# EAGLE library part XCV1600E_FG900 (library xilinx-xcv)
xcv1600e_fg900 edit this description Auto generated by make-symbol-device-package-bsdl.ulp Rev. 26 Source: xcv1600e_fg900.bsd
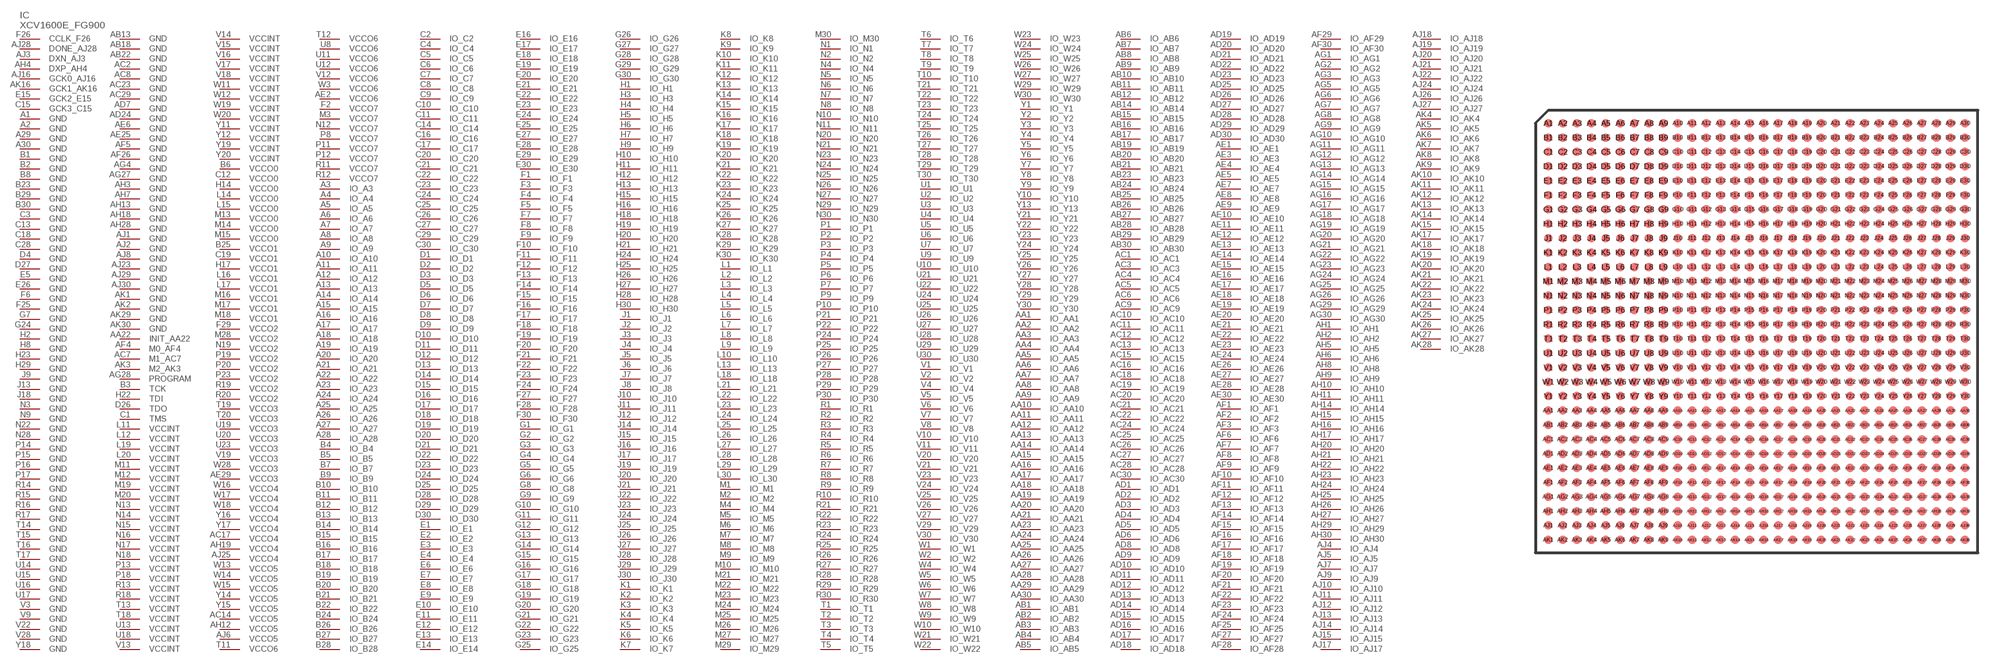
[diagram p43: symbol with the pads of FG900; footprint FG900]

Designator prefix IC

## XCV1600E_FG900 (OC_FARNELL: unknown; OC_NEWARK: unknown)  [FG900]
A1  GND  pwr
A2  GND  pwr
A3  IO_A3
A4  IO_A4
A5  IO_A5
A6  IO_A6
A7  IO_A7
A8  IO_A8
A9  IO_A9
A10  IO_A10
A11  IO_A11
A12  IO_A12
A13  IO_A13
A14  IO_A14
A15  IO_A15
A16  IO_A16
A17  IO_A17
A18  IO_A18
A19  IO_A19
A20  IO_A20
A21  IO_A21
A22  IO_A22
A23  IO_A23
A24  IO_A24
A25  IO_A25
A26  IO_A26
A27  IO_A27
A28  IO_A28
A29  GND  pwr
A30  GND  pwr
AA1  IO_AA1
AA2  IO_AA2
AA3  IO_AA3
AA4  IO_AA4
AA5  IO_AA5
AA6  IO_AA6
AA7  IO_AA7
AA8  IO_AA8
AA9  IO_AA9
AA10  IO_AA10
AA11  IO_AA11
AA12  IO_AA12
AA13  IO_AA13
AA14  IO_AA14
AA15  IO_AA15
AA16  IO_AA16
AA17  IO_AA17
AA18  IO_AA18
AA19  IO_AA19
AA20  IO_AA20
AA21  IO_AA21
AA22  INIT_AA22
AA23  IO_AA23
AA24  IO_AA24
AA25  IO_AA25
AA26  IO_AA26
AA27  IO_AA27
AA28  IO_AA28
AA29  IO_AA29
AA30  IO_AA30
AB1  IO_AB1
AB2  IO_AB2
AB3  IO_AB3
AB4  IO_AB4
AB5  IO_AB5
AB6  IO_AB6
AB7  IO_AB7
AB8  IO_AB8
AB9  IO_AB9
AB10  IO_AB10
AB11  IO_AB11
AB12  IO_AB12
AB13  GND  pwr
AB14  IO_AB14
AB15  IO_AB15
AB16  IO_AB16
AB17  IO_AB17
AB18  GND  pwr
AB19  IO_AB19
AB20  IO_AB20
AB21  IO_AB21
AB22  GND  pwr
AB23  IO_AB23
AB24  IO_AB24
AB25  IO_AB25
AB26  IO_AB26
AB27  IO_AB27
AB28  IO_AB28
AB29  IO_AB29
AB30  IO_AB30
AC1  IO_AC1
AC2  GND  pwr
AC3  IO_AC3
AC4  IO_AC4
AC5  IO_AC5
AC6  IO_AC6
AC7  M1_AC7  in
AC8  GND  pwr
AC9  IO_AC9
AC10  IO_AC10
AC11  IO_AC11
AC12  IO_AC12
AC13  IO_AC13
AC14  VCCO5  pwr
AC15  IO_AC15
AC16  IO_AC16
AC17  VCCO4  pwr
AC18  IO_AC18
AC19  IO_AC19
AC20  IO_AC20
AC21  IO_AC21
AC22  IO_AC22
AC23  GND  pwr
AC24  IO_AC24
AC25  IO_AC25
AC26  IO_AC26
AC27  IO_AC27
AC28  IO_AC28
AC29  GND  pwr
AC30  IO_AC30
AD1  IO_AD1
AD2  IO_AD2
AD3  IO_AD3
AD4  IO_AD4
AD5  IO_AD5
AD6  IO_AD6
AD7  GND  pwr
AD8  IO_AD8
AD9  IO_AD9
AD10  IO_AD10
AD11  IO_AD11
AD12  IO_AD12
AD13  IO_AD13
AD14  IO_AD14
AD15  IO_AD15
AD16  IO_AD16
AD17  IO_AD17
AD18  IO_AD18
AD19  IO_AD19
AD20  IO_AD20
AD21  IO_AD21
AD22  IO_AD22
AD23  IO_AD23
AD24  GND  pwr
AD25  IO_AD25
AD26  IO_AD26
AD27  IO_AD27
AD28  IO_AD28
AD29  IO_AD29
AD30  IO_AD30
AE1  IO_AE1
AE2  VCCO6  pwr
AE3  IO_AE3
AE4  IO_AE4
AE5  IO_AE5
AE6  GND  pwr
AE7  IO_AE7
AE8  IO_AE8
AE9  IO_AE9
AE10  IO_AE10
AE11  IO_AE11
AE12  IO_AE12
AE13  IO_AE13
AE14  IO_AE14
AE15  IO_AE15
AE16  IO_AE16
AE17  IO_AE17
AE18  IO_AE18
AE19  IO_AE19
AE20  IO_AE20
AE21  IO_AE21
AE22  IO_AE22
AE23  IO_AE23
AE24  IO_AE24
AE25  GND  pwr
AE26  IO_AE26
AE27  IO_AE27
AE28  IO_AE28
AE29  VCCO3  pwr
AE30  IO_AE30
AF1  IO_AF1
AF2  IO_AF2
AF3  IO_AF3
AF4  M0_AF4  in
AF5  GND  pwr
AF6  IO_AF6
AF7  IO_AF7
AF8  IO_AF8
AF9  IO_AF9
AF10  IO_AF10
AF11  IO_AF11
AF12  IO_AF12
AF13  IO_AF13
AF14  IO_AF14
AF15  IO_AF15
AF16  IO_AF16
AF17  IO_AF17
AF18  IO_AF18
AF19  IO_AF19
AF20  IO_AF20
AF21  IO_AF21
AF22  IO_AF22
AF23  IO_AF23
AF24  IO_AF24
AF25  IO_AF25
AF26  GND  pwr
AF27  IO_AF27
AF28  IO_AF28
AF29  IO_AF29
AF30  IO_AF30
AG1  IO_AG1
AG2  IO_AG2
AG3  IO_AG3
AG4  GND  pwr
AG5  IO_AG5
AG6  IO_AG6
AG7  IO_AG7
AG8  IO_AG8
AG9  IO_AG9
AG10  IO_AG10
AG11  IO_AG11
AG12  IO_AG12
AG13  IO_AG13
AG14  IO_AG14
AG15  IO_AG15
AG16  IO_AG16
AG17  IO_AG17
AG18  IO_AG18
AG19  IO_AG19
AG20  IO_AG20
AG21  IO_AG21
AG22  IO_AG22
AG23  IO_AG23
AG24  IO_AG24
AG25  IO_AG25
AG26  IO_AG26
AG27  GND  pwr
AG28  PROGRAM  in
AG29  IO_AG29
AG30  IO_AG30
AH1  IO_AH1
AH2  IO_AH2
AH3  GND  pwr
AH4  DXP_AH4  pas
AH5  IO_AH5
AH6  IO_AH6
AH7  GND  pwr
AH8  IO_AH8
AH9  IO_AH9
AH10  IO_AH10
AH11  IO_AH11
AH12  VCCO5  pwr
AH13  GND  pwr
AH14  IO_AH14
AH15  IO_AH15
AH16  IO_AH16
AH17  IO_AH17
AH18  GND  pwr
AH19  VCCO4  pwr
AH20  IO_AH20
AH21  IO_AH21
AH22  IO_AH22
AH23  IO_AH23
AH24  IO_AH24
AH25  IO_AH25
AH26  IO_AH26
AH27  IO_AH27
AH28  GND  pwr
AH29  IO_AH29
AH30  IO_AH30
AJ1  GND  pwr
AJ2  GND  pwr
AJ3  DXN_AJ3  pas
AJ4  IO_AJ4
AJ5  IO_AJ5
AJ6  VCCO5  pwr
AJ7  IO_AJ7
AJ8  GND  pwr
AJ9  IO_AJ9
AJ10  IO_AJ10
AJ11  IO_AJ11
AJ12  IO_AJ12
AJ13  IO_AJ13
AJ14  IO_AJ14
AJ15  IO_AJ15
AJ16  GCK0_AJ16  in
AJ17  IO_AJ17
AJ18  IO_AJ18
AJ19  IO_AJ19
AJ20  IO_AJ20
AJ21  IO_AJ21
AJ22  IO_AJ22
AJ23  GND  pwr
AJ24  IO_AJ24
AJ25  VCCO4  pwr
AJ26  IO_AJ26
AJ27  IO_AJ27
AJ28  DONE_AJ28
AJ29  GND  pwr
AJ30  GND  pwr
AK1  GND  pwr
AK2  GND  pwr
AK3  M2_AK3  in
AK4  IO_AK4
AK5  IO_AK5
AK6  IO_AK6
AK7  IO_AK7
AK8  IO_AK8
AK9  IO_AK9
AK10  IO_AK10
AK11  IO_AK11
AK12  IO_AK12
AK13  IO_AK13
AK14  IO_AK14
AK15  IO_AK15
AK16  GCK1_AK16  in
AK17  IO_AK17
AK18  IO_AK18
AK19  IO_AK19
AK20  IO_AK20
AK21  IO_AK21
AK22  IO_AK22
AK23  IO_AK23
AK24  IO_AK24
AK25  IO_AK25
AK26  IO_AK26
AK27  IO_AK27
AK28  IO_AK28
AK29  GND  pwr
AK30  GND  pwr
B1  GND  pwr
B2  GND  pwr
B3  TCK  in
B4  IO_B4
B5  IO_B5
B6  VCCO0  pwr
B7  IO_B7
B8  GND  pwr
B9  IO_B9
B10  IO_B10
B11  IO_B11
B12  IO_B12
B13  IO_B13
B14  IO_B14
B15  IO_B15
B16  IO_B16
B17  IO_B17
B18  IO_B18
B19  IO_B19
B20  IO_B20
B21  IO_B21
B22  IO_B22
B23  GND  pwr
B24  IO_B24
B25  VCCO1  pwr
B26  IO_B26
B27  IO_B27
B28  IO_B28
B29  GND  pwr
B30  GND  pwr
C1  TMS  in
C2  IO_C2
C3  GND  pwr
C4  IO_C4
C5  IO_C5
C6  IO_C6
C7  IO_C7
C8  IO_C8
C9  IO_C9
C10  IO_C10
C11  IO_C11
C12  VCCO0  pwr
C13  GND  pwr
C14  IO_C14
C15  GCK3_C15  in
C16  IO_C16
C17  IO_C17
C18  GND  pwr
C19  VCCO1  pwr
C20  IO_C20
C21  IO_C21
C22  IO_C22
C23  IO_C23
C24  IO_C24
C25  IO_C25
C26  IO_C26
C27  IO_C27
C28  GND  pwr
C29  IO_C29
C30  IO_C30
D1  IO_D1
D2  IO_D2
D3  IO_D3
D4  GND  pwr
D5  IO_D5
D6  IO_D6
D7  IO_D7
D8  IO_D8
D9  IO_D9
D10  IO_D10
D11  IO_D11
D12  IO_D12
D13  IO_D13
D14  IO_D14
D15  IO_D15
D16  IO_D16
D17  IO_D17
D18  IO_D18
D19  IO_D19
D20  IO_D20
D21  IO_D21
D22  IO_D22
D23  IO_D23
D24  IO_D24
D25  IO_D25
D26  TDO  out
D27  GND  pwr
D28  IO_D28
D29  IO_D29
D30  IO_D30
E1  IO_E1
E2  IO_E2
E3  IO_E3
E4  IO_E4
E5  GND  pwr
E6  IO_E6
E7  IO_E7
E8  IO_E8
E9  IO_E9
E10  IO_E10
E11  IO_E11
E12  IO_E12
E13  IO_E13
E14  IO_E14
E15  GCK2_E15  in
E16  IO_E16
E17  IO_E17
E18  IO_E18
E19  IO_E19
E20  IO_E20
E21  IO_E21
E22  IO_E22
E23  IO_E23
E24  IO_E24
E25  IO_E25
E26  GND  pwr
E27  IO_E27
E28  IO_E28
E29  IO_E29
E30  IO_E30
F1  IO_F1
F2  VCCO7  pwr
F3  IO_F3
F4  IO_F4
F5  IO_F5
F6  GND  pwr
F7  IO_F7
F8  IO_F8
F9  IO_F9
F10  IO_F10
F11  IO_F11
F12  IO_F12
F13  IO_F13
F14  IO_F14
F15  IO_F15
F16  IO_F16
F17  IO_F17
F18  IO_F18
F19  IO_F19
F20  IO_F20
F21  IO_F21
F22  IO_F22
F23  IO_F23
F24  IO_F24
F25  GND  pwr
F26  CCLK_F26
F27  IO_F27
F28  IO_F28
F29  VCCO2  pwr
F30  IO_F30
G1  IO_G1
G2  IO_G2
G3  IO_G3
G4  IO_G4
G5  IO_G5
G6  IO_G6
G7  GND  pwr
G8  IO_G8
G9  IO_G9
G10  IO_G10
G11  IO_G11
G12  IO_G12
G13  IO_G13
G14  IO_G14
G15  IO_G15
G16  IO_G16
G17  IO_G17
G18  IO_G18
G19  IO_G19
G20  IO_G20
G21  IO_G21
G22  IO_G22
G23  IO_G23
G24  GND  pwr
G25  IO_G25
G26  IO_G26
G27  IO_G27
G28  IO_G28
G29  IO_G29
G30  IO_G30
H1  IO_H1
H2  GND  pwr
H3  IO_H3
H4  IO_H4
H5  IO_H5
H6  IO_H6
H7  IO_H7
H8  GND  pwr
H9  IO_H9
H10  IO_H10
H11  IO_H11
H12  IO_H12
H13  IO_H13
H14  VCCO0  pwr
H15  IO_H15
H16  IO_H16
H17  VCCO1  pwr
H18  IO_H18
H19  IO_H19
H20  IO_H20
H21  IO_H21
H22  TDI  in
H23  GND  pwr
H24  IO_H24
H25  IO_H25
H26  IO_H26
H27  IO_H27
H28  IO_H28
H29  GND  pwr
H30  IO_H30
J1  IO_J1
J2  IO_J2
J3  IO_J3
J4  IO_J4
J5  IO_J5
J6  IO_J6
J7  IO_J7
J8  IO_J8
J9  GND  pwr
J10  IO_J10
J11  IO_J11
J12  IO_J12
J13  GND  pwr
J14  IO_J14
J15  IO_J15
J16  IO_J16
J17  IO_J17
J18  GND  pwr
J19  IO_J19
J20  IO_J20
J21  IO_J21
J22  IO_J22
J23  IO_J23
J24  IO_J24
J25  IO_J25
J26  IO_J26
J27  IO_J27
J28  IO_J28
J29  IO_J29
J30  IO_J30
K1  IO_K1
K2  IO_K2
K3  IO_K3
K4  IO_K4
K5  IO_K5
K6  IO_K6
K7  IO_K7
K8  IO_K8
K9  IO_K9
K10  IO_K10
K11  IO_K11
K12  IO_K12
K13  IO_K13
K14  IO_K14
K15  IO_K15
K16  IO_K16
K17  IO_K17
K18  IO_K18
K19  IO_K19
K20  IO_K20
K21  IO_K21
K22  IO_K22
K23  IO_K23
K24  IO_K24
K25  IO_K25
K26  IO_K26
K27  IO_K27
K28  IO_K28
K29  IO_K29
K30  IO_K30
L1  IO_L1
L2  IO_L2
L3  IO_L3
L4  IO_L4
L5  IO_L5
L6  IO_L6
L7  IO_L7
L8  IO_L8
L9  IO_L9
L10  IO_L10
L11  VCCINT  pwr
L12  VCCINT  pwr
L13  IO_L13
L14  VCCO0  pwr
L15  VCCO0  pwr
L16  VCCO1  pwr
L17  VCCO1  pwr
L18  IO_L18
L19  VCCINT  pwr
L20  VCCINT  pwr
L21  IO_L21
L22  IO_L22
L23  IO_L23
L24  IO_L24
L25  IO_L25
L26  IO_L26
L27  IO_L27
L28  IO_L28
L29  IO_L29
L30  IO_L30
M1  IO_M1
M2  IO_M2
M3  VCCO7  pwr
M4  IO_M4
M5  IO_M5
M6  IO_M6
M7  IO_M7
M8  IO_M8
M9  IO_M9
M10  IO_M10
M11  VCCINT  pwr
M12  VCCINT  pwr
M13  VCCO0  pwr
M14  VCCO0  pwr
M15  VCCO0  pwr
M16  VCCO1  pwr
M17  VCCO1  pwr
M18  VCCO1  pwr
M19  VCCINT  pwr
M20  VCCINT  pwr
M21  IO_M21
M22  IO_M22
M23  IO_M23
M24  IO_M24
M25  IO_M25
M26  IO_M26
M27  IO_M27
M28  VCCO2  pwr
M29  IO_M29
M30  IO_M30
N1  IO_N1
N2  IO_N2
N3  GND  pwr
N4  IO_N4
N5  IO_N5
N6  IO_N6
N7  IO_N7
N8  IO_N8
N9  GND  pwr
N10  IO_N10
N11  IO_N11
N12  VCCO7  pwr
N13  VCCINT  pwr
N14  VCCINT  pwr
N15  VCCINT  pwr
N16  VCCINT  pwr
N17  VCCINT  pwr
N18  VCCINT  pwr
N19  VCCO2  pwr
N20  IO_N20
N21  IO_N21
N22  GND  pwr
N23  IO_N23
N24  IO_N24
N25  IO_N25
N26  IO_N26
N27  IO_N27
N28  GND  pwr
N29  IO_N29
N30  IO_N30
P1  IO_P1
P2  IO_P2
P3  IO_P3
P4  IO_P4
P5  IO_P5
P6  IO_P6
P7  IO_P7
P8  VCCO7  pwr
P9  IO_P9
P10  IO_P10
P11  VCCO7  pwr
P12  VCCO7  pwr
P13  VCCINT  pwr
P14  GND  pwr
P15  GND  pwr
P16  GND  pwr
P17  GND  pwr
P18  VCCINT  pwr
P19  VCCO2  pwr
P20  VCCO2  pwr
P21  IO_P21
P22  IO_P22
P23  VCCO2  pwr
P24  IO_P24
P25  IO_P25
P26  IO_P26
P27  IO_P27
P28  IO_P28
P29  IO_P29
P30  IO_P30
R1  IO_R1
R2  IO_R2
R3  IO_R3
R4  IO_R4
R5  IO_R5
R6  IO_R6
R7  IO_R7
R8  IO_R8
R9  IO_R9
R10  IO_R10
R11  VCCO7  pwr
R12  VCCO7  pwr
R13  VCCINT  pwr
R14  GND  pwr
R15  GND  pwr
R16  GND  pwr
R17  GND  pwr
R18  VCCINT  pwr
R19  VCCO2  pwr
R20  VCCO2  pwr
R21  IO_R21
R22  IO_R22
R23  IO_R23
R24  IO_R24
R25  IO_R25
R26  IO_R26
R27  IO_R27
R28  IO_R28
R29  IO_R29
R30  IO_R30
T1  IO_T1
T2  IO_T2
T3  IO_T3
T4  IO_T4
T5  IO_T5
T6  IO_T6
T7  IO_T7
T8  IO_T8
T9  IO_T9
T10  IO_T10
T11  VCCO6  pwr
T12  VCCO6  pwr
T13  VCCINT  pwr
T14  GND  pwr
T15  GND  pwr
T16  GND  pwr
T17  GND  pwr
T18  VCCINT  pwr
T19  VCCO3  pwr
T20  VCCO3  pwr
T21  IO_T21
T22  IO_T22
T23  IO_T23
T24  IO_T24
T25  IO_T25
T26  IO_T26
T27  IO_T27
T28  IO_T28
T29  IO_T29
T30  IO_T30
U1  IO_U1
U2  IO_U2
U3  IO_U3
U4  IO_U4
U5  IO_U5
U6  IO_U6
U7  IO_U7
U8  VCCO6  pwr
U9  IO_U9
U10  IO_U10
U11  VCCO6  pwr
U12  VCCO6  pwr
U13  VCCINT  pwr
U14  GND  pwr
U15  GND  pwr
U16  GND  pwr
U17  GND  pwr
U18  VCCINT  pwr
U19  VCCO3  pwr
U20  VCCO3  pwr
U21  IO_U21
U22  IO_U22
U23  VCCO3  pwr
U24  IO_U24
U25  IO_U25
U26  IO_U26
U27  IO_U27
U28  IO_U28
U29  IO_U29
U30  IO_U30
V1  IO_V1
V2  IO_V2
V3  GND  pwr
V4  IO_V4
V5  IO_V5
V6  IO_V6
V7  IO_V7
V8  IO_V8
V9  GND  pwr
V10  IO_V10
V11  IO_V11
V12  VCCO6  pwr
V13  VCCINT  pwr
V14  VCCINT  pwr
V15  VCCINT  pwr
V16  VCCINT  pwr
V17  VCCINT  pwr
V18  VCCINT  pwr
V19  VCCO3  pwr
V20  IO_V20
V21  IO_V21
V22  GND  pwr
V23  IO_V23
V24  IO_V24
V25  IO_V25
V26  IO_V26
V27  IO_V27
V28  GND  pwr
V29  IO_V29
V30  IO_V30
W1  IO_W1
W2  IO_W2
W3  VCCO6  pwr
W4  IO_W4
W5  IO_W5
W6  IO_W6
W7  IO_W7
W8  IO_W8
W9  IO_W9
W10  IO_W10
W11  VCCINT  pwr
W12  VCCINT  pwr
W13  VCCO5  pwr
W14  VCCO5  pwr
W15  VCCO5  pwr
W16  VCCO4  pwr
W17  VCCO4  pwr
W18  VCCO4  pwr
W19  VCCINT  pwr
W20  VCCINT  pwr
W21  IO_W21
W22  IO_W22
W23  IO_W23
W24  IO_W24
W25  IO_W25
W26  IO_W26
W27  IO_W27
W28  VCCO3  pwr
W29  IO_W29
W30  IO_W30
Y1  IO_Y1
Y2  IO_Y2
Y3  IO_Y3
Y4  IO_Y4
Y5  IO_Y5
Y6  IO_Y6
Y7  IO_Y7
Y8  IO_Y8
Y9  IO_Y9
Y10  IO_Y10
Y11  VCCINT  pwr
Y12  VCCINT  pwr
Y13  IO_Y13
Y14  VCCO5  pwr
Y15  VCCO5  pwr
Y16  VCCO4  pwr
Y17  VCCO4  pwr
Y18  GND  pwr
Y19  VCCINT  pwr
Y20  VCCINT  pwr
Y21  IO_Y21
Y22  IO_Y22
Y23  IO_Y23
Y24  IO_Y24
Y25  IO_Y25
Y26  IO_Y26
Y27  IO_Y27
Y28  IO_Y28
Y29  IO_Y29
Y30  IO_Y30

## Footprint FG900 (pad centres in mm)
xcv1000e_fg900_1532 edit this description Auto generated by make-symbol-device-package-bsdl.ulp Rev. 26 Source: xcv1000e_fg900_1532.bsd
smd 0.6 x 0.6: A1 -14.5,14.5; A2 -13.5,14.5; A3 -12.5,14.5; A4 -11.5,14.5; A5 -10.5,14.5; A6 -9.5,14.5; A7 -8.5,14.5; A8 -7.5,14.5; A9 -6.5,14.5; A10 -5.5,14.5; A11 -4.5,14.5; A12 -3.5,14.5; A13 -2.5,14.5; A14 -1.5,14.5; A15 -0.5,14.5; A16 0.5,14.5; A17 1.5,14.5; A18 2.5,14.5; A19 3.5,14.5; A20 4.5,14.5; A21 5.5,14.5; A22 6.5,14.5; A23 7.5,14.5; A24 8.5,14.5; A25 9.5,14.5; A26 10.5,14.5; A27 11.5,14.5; A28 12.5,14.5; A29 13.5,14.5; A30 14.5,14.5; AA1 -14.5,-5.5; AA2 -13.5,-5.5; AA3 -12.5,-5.5; AA4 -11.5,-5.5; AA5 -10.5,-5.5; AA6 -9.5,-5.5; AA7 -8.5,-5.5; AA8 -7.5,-5.5; AA9 -6.5,-5.5; AA10 -5.5,-5.5; AA11 -4.5,-5.5; AA12 -3.5,-5.5; AA13 -2.5,-5.5; AA14 -1.5,-5.5; AA15 -0.5,-5.5; AA16 0.5,-5.5; AA17 1.5,-5.5; AA18 2.5,-5.5; AA19 3.5,-5.5; AA20 4.5,-5.5; AA21 5.5,-5.5; AA22 6.5,-5.5; AA23 7.5,-5.5; AA24 8.5,-5.5; AA25 9.5,-5.5; AA26 10.5,-5.5; AA27 11.5,-5.5; AA28 12.5,-5.5; AA29 13.5,-5.5; AA30 14.5,-5.5; AB1 -14.5,-6.5; AB2 -13.5,-6.5; AB3 -12.5,-6.5; AB4 -11.5,-6.5; AB5 -10.5,-6.5; AB6 -9.5,-6.5; AB7 -8.5,-6.5; AB8 -7.5,-6.5; AB9 -6.5,-6.5; AB10 -5.5,-6.5; AB11 -4.5,-6.5; AB12 -3.5,-6.5; AB13 -2.5,-6.5; AB14 -1.5,-6.5; AB15 -0.5,-6.5; AB16 0.5,-6.5; AB17 1.5,-6.5; AB18 2.5,-6.5; AB19 3.5,-6.5; AB20 4.5,-6.5; AB21 5.5,-6.5; AB22 6.5,-6.5; AB23 7.5,-6.5; AB24 8.5,-6.5; AB25 9.5,-6.5; AB26 10.5,-6.5; AB27 11.5,-6.5; AB28 12.5,-6.5; AB29 13.5,-6.5; AB30 14.5,-6.5; AC1 -14.5,-7.5; AC2 -13.5,-7.5; AC3 -12.5,-7.5; AC4 -11.5,-7.5; AC5 -10.5,-7.5; AC6 -9.5,-7.5; AC7 -8.5,-7.5; AC8 -7.5,-7.5; AC9 -6.5,-7.5; AC10 -5.5,-7.5; AC11 -4.5,-7.5; AC12 -3.5,-7.5; AC13 -2.5,-7.5; AC14 -1.5,-7.5; AC15 -0.5,-7.5; AC16 0.5,-7.5; AC17 1.5,-7.5; AC18 2.5,-7.5; AC19 3.5,-7.5; AC20 4.5,-7.5; AC21 5.5,-7.5; AC22 6.5,-7.5; AC23 7.5,-7.5; AC24 8.5,-7.5; AC25 9.5,-7.5; AC26 10.5,-7.5; AC27 11.5,-7.5; AC28 12.5,-7.5; AC29 13.5,-7.5; AC30 14.5,-7.5; AD1 -14.5,-8.5; AD2 -13.5,-8.5; AD3 -12.5,-8.5; AD4 -11.5,-8.5; AD5 -10.5,-8.5; AD6 -9.5,-8.5; AD7 -8.5,-8.5; AD8 -7.5,-8.5; AD9 -6.5,-8.5; AD10 -5.5,-8.5; AD11 -4.5,-8.5; AD12 -3.5,-8.5; AD13 -2.5,-8.5; AD14 -1.5,-8.5; AD15 -0.5,-8.5; AD16 0.5,-8.5; AD17 1.5,-8.5; AD18 2.5,-8.5; AD19 3.5,-8.5; AD20 4.5,-8.5; AD21 5.5,-8.5; AD22 6.5,-8.5; AD23 7.5,-8.5; AD24 8.5,-8.5; AD25 9.5,-8.5; AD26 10.5,-8.5; AD27 11.5,-8.5; AD28 12.5,-8.5; AD29 13.5,-8.5; AD30 14.5,-8.5; AE1 -14.5,-9.5; AE2 -13.5,-9.5; AE3 -12.5,-9.5; AE4 -11.5,-9.5; AE5 -10.5,-9.5; AE6 -9.5,-9.5; AE7 -8.5,-9.5; AE8 -7.5,-9.5; AE9 -6.5,-9.5; AE10 -5.5,-9.5; AE11 -4.5,-9.5; AE12 -3.5,-9.5; AE13 -2.5,-9.5; AE14 -1.5,-9.5; AE15 -0.5,-9.5; AE16 0.5,-9.5; AE17 1.5,-9.5; AE18 2.5,-9.5; AE19 3.5,-9.5; AE20 4.5,-9.5; AE21 5.5,-9.5; AE22 6.5,-9.5; AE23 7.5,-9.5; AE24 8.5,-9.5; AE25 9.5,-9.5; AE26 10.5,-9.5; AE27 11.5,-9.5; AE28 12.5,-9.5; AE29 13.5,-9.5; AE30 14.5,-9.5; AF1 -14.5,-10.5; AF2 -13.5,-10.5; AF3 -12.5,-10.5; AF4 -11.5,-10.5; AF5 -10.5,-10.5; AF6 -9.5,-10.5; AF7 -8.5,-10.5; AF8 -7.5,-10.5; AF9 -6.5,-10.5; AF10 -5.5,-10.5; AF11 -4.5,-10.5; AF12 -3.5,-10.5; AF13 -2.5,-10.5; AF14 -1.5,-10.5; AF15 -0.5,-10.5; AF16 0.5,-10.5; AF17 1.5,-10.5; AF18 2.5,-10.5; AF19 3.5,-10.5; AF20 4.5,-10.5; AF21 5.5,-10.5; AF22 6.5,-10.5; AF23 7.5,-10.5; AF24 8.5,-10.5; AF25 9.5,-10.5; AF26 10.5,-10.5; AF27 11.5,-10.5; AF28 12.5,-10.5; AF29 13.5,-10.5; AF30 14.5,-10.5; AG1 -14.5,-11.5; AG2 -13.5,-11.5; AG3 -12.5,-11.5; AG4 -11.5,-11.5; AG5 -10.5,-11.5; AG6 -9.5,-11.5; AG7 -8.5,-11.5; AG8 -7.5,-11.5; AG9 -6.5,-11.5; AG10 -5.5,-11.5; AG11 -4.5,-11.5; AG12 -3.5,-11.5; AG13 -2.5,-11.5; AG14 -1.5,-11.5; AG15 -0.5,-11.5; AG16 0.5,-11.5; AG17 1.5,-11.5; AG18 2.5,-11.5; AG19 3.5,-11.5; AG20 4.5,-11.5; AG21 5.5,-11.5; AG22 6.5,-11.5; AG23 7.5,-11.5; AG24 8.5,-11.5; AG25 9.5,-11.5; AG26 10.5,-11.5; AG27 11.5,-11.5; AG28 12.5,-11.5; AG29 13.5,-11.5; AG30 14.5,-11.5; AH1 -14.5,-12.5; AH2 -13.5,-12.5; AH3 -12.5,-12.5; AH4 -11.5,-12.5; AH5 -10.5,-12.5; AH6 -9.5,-12.5; AH7 -8.5,-12.5; AH8 -7.5,-12.5; AH9 -6.5,-12.5; AH10 -5.5,-12.5; AH11 -4.5,-12.5; AH12 -3.5,-12.5; AH13 -2.5,-12.5; AH14 -1.5,-12.5; AH15 -0.5,-12.5; AH16 0.5,-12.5; AH17 1.5,-12.5; AH18 2.5,-12.5; AH19 3.5,-12.5; AH20 4.5,-12.5; AH21 5.5,-12.5; AH22 6.5,-12.5; AH23 7.5,-12.5; AH24 8.5,-12.5; AH25 9.5,-12.5; AH26 10.5,-12.5; AH27 11.5,-12.5; AH28 12.5,-12.5; AH29 13.5,-12.5; AH30 14.5,-12.5; AJ1 -14.5,-13.5; AJ2 -13.5,-13.5; AJ3 -12.5,-13.5; AJ4 -11.5,-13.5; AJ5 -10.5,-13.5; AJ6 -9.5,-13.5; AJ7 -8.5,-13.5; AJ8 -7.5,-13.5; AJ9 -6.5,-13.5; AJ10 -5.5,-13.5; AJ11 -4.5,-13.5; AJ12 -3.5,-13.5; AJ13 -2.5,-13.5; AJ14 -1.5,-13.5; AJ15 -0.5,-13.5; AJ16 0.5,-13.5; AJ17 1.5,-13.5; AJ18 2.5,-13.5; AJ19 3.5,-13.5; AJ20 4.5,-13.5; AJ21 5.5,-13.5; AJ22 6.5,-13.5; AJ23 7.5,-13.5; AJ24 8.5,-13.5; AJ25 9.5,-13.5; AJ26 10.5,-13.5; AJ27 11.5,-13.5; AJ28 12.5,-13.5; AJ29 13.5,-13.5; AJ30 14.5,-13.5; AK1 -14.5,-14.5; AK2 -13.5,-14.5; AK3 -12.5,-14.5; AK4 -11.5,-14.5; AK5 -10.5,-14.5; AK6 -9.5,-14.5; AK7 -8.5,-14.5; AK8 -7.5,-14.5; AK9 -6.5,-14.5; AK10 -5.5,-14.5; AK11 -4.5,-14.5; AK12 -3.5,-14.5; AK13 -2.5,-14.5; AK14 -1.5,-14.5; AK15 -0.5,-14.5; AK16 0.5,-14.5; AK17 1.5,-14.5; AK18 2.5,-14.5; AK19 3.5,-14.5; AK20 4.5,-14.5; AK21 5.5,-14.5; AK22 6.5,-14.5; AK23 7.5,-14.5; AK24 8.5,-14.5; AK25 9.5,-14.5; AK26 10.5,-14.5; AK27 11.5,-14.5; AK28 12.5,-14.5; AK29 13.5,-14.5; AK30 14.5,-14.5; B1 -14.5,13.5; B2 -13.5,13.5; B3 -12.5,13.5; B4 -11.5,13.5; B5 -10.5,13.5; B6 -9.5,13.5; B7 -8.5,13.5; B8 -7.5,13.5; B9 -6.5,13.5; B10 -5.5,13.5; B11 -4.5,13.5; B12 -3.5,13.5; B13 -2.5,13.5; B14 -1.5,13.5; B15 -0.5,13.5; B16 0.5,13.5; B17 1.5,13.5; B18 2.5,13.5; B19 3.5,13.5; B20 4.5,13.5; B21 5.5,13.5; B22 6.5,13.5; B23 7.5,13.5; B24 8.5,13.5; B25 9.5,13.5; B26 10.5,13.5; B27 11.5,13.5; B28 12.5,13.5; B29 13.5,13.5; B30 14.5,13.5; C1 -14.5,12.5; C2 -13.5,12.5; C3 -12.5,12.5; C4 -11.5,12.5; C5 -10.5,12.5; C6 -9.5,12.5; C7 -8.5,12.5; C8 -7.5,12.5; C9 -6.5,12.5; C10 -5.5,12.5; C11 -4.5,12.5; C12 -3.5,12.5; C13 -2.5,12.5; C14 -1.5,12.5; C15 -0.5,12.5; C16 0.5,12.5; C17 1.5,12.5; C18 2.5,12.5; C19 3.5,12.5; C20 4.5,12.5; C21 5.5,12.5; C22 6.5,12.5; C23 7.5,12.5; C24 8.5,12.5; C25 9.5,12.5; C26 10.5,12.5; C27 11.5,12.5; C28 12.5,12.5; C29 13.5,12.5; C30 14.5,12.5; D1 -14.5,11.5; D2 -13.5,11.5; D3 -12.5,11.5; D4 -11.5,11.5; D5 -10.5,11.5; D6 -9.5,11.5; D7 -8.5,11.5; D8 -7.5,11.5; D9 -6.5,11.5; D10 -5.5,11.5; D11 -4.5,11.5; D12 -3.5,11.5; D13 -2.5,11.5; D14 -1.5,11.5; D15 -0.5,11.5; D16 0.5,11.5; D17 1.5,11.5; D18 2.5,11.5; D19 3.5,11.5; D20 4.5,11.5; D21 5.5,11.5; D22 6.5,11.5; D23 7.5,11.5; D24 8.5,11.5; D25 9.5,11.5; D26 10.5,11.5; D27 11.5,11.5; D28 12.5,11.5; D29 13.5,11.5; D30 14.5,11.5; E1 -14.5,10.5; E2 -13.5,10.5; E3 -12.5,10.5; E4 -11.5,10.5; E5 -10.5,10.5; E6 -9.5,10.5; E7 -8.5,10.5; E8 -7.5,10.5; E9 -6.5,10.5; E10 -5.5,10.5; E11 -4.5,10.5; E12 -3.5,10.5; E13 -2.5,10.5; E14 -1.5,10.5; E15 -0.5,10.5; E16 0.5,10.5; E17 1.5,10.5; E18 2.5,10.5; E19 3.5,10.5; E20 4.5,10.5; E21 5.5,10.5; E22 6.5,10.5; E23 7.5,10.5; E24 8.5,10.5; E25 9.5,10.5; E26 10.5,10.5; E27 11.5,10.5; E28 12.5,10.5; E29 13.5,10.5; E30 14.5,10.5; F1 -14.5,9.5; F2 -13.5,9.5; F3 -12.5,9.5; F4 -11.5,9.5; F5 -10.5,9.5; F6 -9.5,9.5; F7 -8.5,9.5; F8 -7.5,9.5; F9 -6.5,9.5; F10 -5.5,9.5; F11 -4.5,9.5; F12 -3.5,9.5; F13 -2.5,9.5; F14 -1.5,9.5; F15 -0.5,9.5; F16 0.5,9.5; F17 1.5,9.5; F18 2.5,9.5; F19 3.5,9.5; F20 4.5,9.5; F21 5.5,9.5; F22 6.5,9.5; F23 7.5,9.5; F24 8.5,9.5; F25 9.5,9.5; F26 10.5,9.5; F27 11.5,9.5; F28 12.5,9.5; F29 13.5,9.5; F30 14.5,9.5; G1 -14.5,8.5; G2 -13.5,8.5; G3 -12.5,8.5; G4 -11.5,8.5; G5 -10.5,8.5; G6 -9.5,8.5; G7 -8.5,8.5; G8 -7.5,8.5; G9 -6.5,8.5; G10 -5.5,8.5; G11 -4.5,8.5; G12 -3.5,8.5; G13 -2.5,8.5; G14 -1.5,8.5; G15 -0.5,8.5; G16 0.5,8.5; G17 1.5,8.5; G18 2.5,8.5; G19 3.5,8.5; G20 4.5,8.5; G21 5.5,8.5; G22 6.5,8.5; G23 7.5,8.5; G24 8.5,8.5; G25 9.5,8.5; G26 10.5,8.5; G27 11.5,8.5; G28 12.5,8.5; G29 13.5,8.5; G30 14.5,8.5; H1 -14.5,7.5; H2 -13.5,7.5; H3 -12.5,7.5; H4 -11.5,7.5; H5 -10.5,7.5; H6 -9.5,7.5; H7 -8.5,7.5; H8 -7.5,7.5; H9 -6.5,7.5; H10 -5.5,7.5; H11 -4.5,7.5; H12 -3.5,7.5; H13 -2.5,7.5; H14 -1.5,7.5; H15 -0.5,7.5; H16 0.5,7.5; H17 1.5,7.5; H18 2.5,7.5; H19 3.5,7.5; H20 4.5,7.5; H21 5.5,7.5; H22 6.5,7.5; H23 7.5,7.5; H24 8.5,7.5; H25 9.5,7.5; H26 10.5,7.5; H27 11.5,7.5; H28 12.5,7.5; H29 13.5,7.5; H30 14.5,7.5; J1 -14.5,6.5; J2 -13.5,6.5; J3 -12.5,6.5; J4 -11.5,6.5; J5 -10.5,6.5; J6 -9.5,6.5; J7 -8.5,6.5; J8 -7.5,6.5; J9 -6.5,6.5; J10 -5.5,6.5; J11 -4.5,6.5; J12 -3.5,6.5; J13 -2.5,6.5; J14 -1.5,6.5; J15 -0.5,6.5; J16 0.5,6.5; J17 1.5,6.5; J18 2.5,6.5; J19 3.5,6.5; J20 4.5,6.5; J21 5.5,6.5; J22 6.5,6.5; J23 7.5,6.5; J24 8.5,6.5; J25 9.5,6.5; J26 10.5,6.5; J27 11.5,6.5; J28 12.5,6.5; J29 13.5,6.5; J30 14.5,6.5; K1 -14.5,5.5; K2 -13.5,5.5; K3 -12.5,5.5; K4 -11.5,5.5; K5 -10.5,5.5; K6 -9.5,5.5; K7 -8.5,5.5; K8 -7.5,5.5; K9 -6.5,5.5; K10 -5.5,5.5; K11 -4.5,5.5; K12 -3.5,5.5; K13 -2.5,5.5; K14 -1.5,5.5; K15 -0.5,5.5; K16 0.5,5.5; K17 1.5,5.5; K18 2.5,5.5; K19 3.5,5.5; K20 4.5,5.5; K21 5.5,5.5; K22 6.5,5.5; K23 7.5,5.5; K24 8.5,5.5; K25 9.5,5.5; K26 10.5,5.5; K27 11.5,5.5; K28 12.5,5.5; K29 13.5,5.5; K30 14.5,5.5; L1 -14.5,4.5; L2 -13.5,4.5; L3 -12.5,4.5; L4 -11.5,4.5; L5 -10.5,4.5; L6 -9.5,4.5; L7 -8.5,4.5; L8 -7.5,4.5; L9 -6.5,4.5; L10 -5.5,4.5; L11 -4.5,4.5; L12 -3.5,4.5; L13 -2.5,4.5; L14 -1.5,4.5; L15 -0.5,4.5; L16 0.5,4.5; L17 1.5,4.5; L18 2.5,4.5; L19 3.5,4.5; L20 4.5,4.5; L21 5.5,4.5; L22 6.5,4.5; L23 7.5,4.5; L24 8.5,4.5; L25 9.5,4.5; L26 10.5,4.5; L27 11.5,4.5; L28 12.5,4.5; L29 13.5,4.5; L30 14.5,4.5; M1 -14.5,3.5; M2 -13.5,3.5; M3 -12.5,3.5; M4 -11.5,3.5; M5 -10.5,3.5; M6 -9.5,3.5; M7 -8.5,3.5; M8 -7.5,3.5; M9 -6.5,3.5; M10 -5.5,3.5; M11 -4.5,3.5; M12 -3.5,3.5; M13 -2.5,3.5; M14 -1.5,3.5; M15 -0.5,3.5; M16 0.5,3.5; M17 1.5,3.5; M18 2.5,3.5; M19 3.5,3.5; M20 4.5,3.5; M21 5.5,3.5; M22 6.5,3.5; M23 7.5,3.5; M24 8.5,3.5; M25 9.5,3.5; M26 10.5,3.5; M27 11.5,3.5; M28 12.5,3.5; M29 13.5,3.5; M30 14.5,3.5; N1 -14.5,2.5; N2 -13.5,2.5; N3 -12.5,2.5; N4 -11.5,2.5; N5 -10.5,2.5; N6 -9.5,2.5; N7 -8.5,2.5; N8 -7.5,2.5; N9 -6.5,2.5; N10 -5.5,2.5; N11 -4.5,2.5; N12 -3.5,2.5; N13 -2.5,2.5; N14 -1.5,2.5; N15 -0.5,2.5; N16 0.5,2.5; N17 1.5,2.5; N18 2.5,2.5; N19 3.5,2.5; N20 4.5,2.5; N21 5.5,2.5; N22 6.5,2.5; N23 7.5,2.5; N24 8.5,2.5; N25 9.5,2.5; N26 10.5,2.5; N27 11.5,2.5; N28 12.5,2.5; N29 13.5,2.5; N30 14.5,2.5; P1 -14.5,1.5; P2 -13.5,1.5; P3 -12.5,1.5; P4 -11.5,1.5; P5 -10.5,1.5; P6 -9.5,1.5; P7 -8.5,1.5; P8 -7.5,1.5; P9 -6.5,1.5; P10 -5.5,1.5; P11 -4.5,1.5; P12 -3.5,1.5; P13 -2.5,1.5; P14 -1.5,1.5; P15 -0.5,1.5; P16 0.5,1.5; P17 1.5,1.5; P18 2.5,1.5; P19 3.5,1.5; P20 4.5,1.5; P21 5.5,1.5; P22 6.5,1.5; P23 7.5,1.5; P24 8.5,1.5; P25 9.5,1.5; P26 10.5,1.5; P27 11.5,1.5; P28 12.5,1.5; P29 13.5,1.5; P30 14.5,1.5; R1 -14.5,0.5; R2 -13.5,0.5; R3 -12.5,0.5; R4 -11.5,0.5; R5 -10.5,0.5; R6 -9.5,0.5; R7 -8.5,0.5; R8 -7.5,0.5; R9 -6.5,0.5; R10 -5.5,0.5; R11 -4.5,0.5; R12 -3.5,0.5; R13 -2.5,0.5; R14 -1.5,0.5; R15 -0.5,0.5; R16 0.5,0.5; R17 1.5,0.5; R18 2.5,0.5; R19 3.5,0.5; R20 4.5,0.5; R21 5.5,0.5; R22 6.5,0.5; R23 7.5,0.5; R24 8.5,0.5; R25 9.5,0.5; R26 10.5,0.5; R27 11.5,0.5; R28 12.5,0.5; R29 13.5,0.5; R30 14.5,0.5; T1 -14.5,-0.5; T2 -13.5,-0.5; T3 -12.5,-0.5; T4 -11.5,-0.5; T5 -10.5,-0.5; T6 -9.5,-0.5; T7 -8.5,-0.5; T8 -7.5,-0.5; T9 -6.5,-0.5; T10 -5.5,-0.5; T11 -4.5,-0.5; T12 -3.5,-0.5; T13 -2.5,-0.5; T14 -1.5,-0.5; T15 -0.5,-0.5; T16 0.5,-0.5; T17 1.5,-0.5; T18 2.5,-0.5; T19 3.5,-0.5; T20 4.5,-0.5; T21 5.5,-0.5; T22 6.5,-0.5; T23 7.5,-0.5; T24 8.5,-0.5; T25 9.5,-0.5; T26 10.5,-0.5; T27 11.5,-0.5; T28 12.5,-0.5; T29 13.5,-0.5; T30 14.5,-0.5; U1 -14.5,-1.5; U2 -13.5,-1.5; U3 -12.5,-1.5; U4 -11.5,-1.5; U5 -10.5,-1.5; U6 -9.5,-1.5; U7 -8.5,-1.5; U8 -7.5,-1.5; U9 -6.5,-1.5; U10 -5.5,-1.5; U11 -4.5,-1.5; U12 -3.5,-1.5; U13 -2.5,-1.5; U14 -1.5,-1.5; U15 -0.5,-1.5; U16 0.5,-1.5; U17 1.5,-1.5; U18 2.5,-1.5; U19 3.5,-1.5; U20 4.5,-1.5; U21 5.5,-1.5; U22 6.5,-1.5; U23 7.5,-1.5; U24 8.5,-1.5; U25 9.5,-1.5; U26 10.5,-1.5; U27 11.5,-1.5; U28 12.5,-1.5; U29 13.5,-1.5; U30 14.5,-1.5; V1 -14.5,-2.5; V2 -13.5,-2.5; V3 -12.5,-2.5; V4 -11.5,-2.5; V5 -10.5,-2.5; V6 -9.5,-2.5; V7 -8.5,-2.5; V8 -7.5,-2.5; V9 -6.5,-2.5; V10 -5.5,-2.5; V11 -4.5,-2.5; V12 -3.5,-2.5; V13 -2.5,-2.5; V14 -1.5,-2.5; V15 -0.5,-2.5; V16 0.5,-2.5; V17 1.5,-2.5; V18 2.5,-2.5; V19 3.5,-2.5; V20 4.5,-2.5; V21 5.5,-2.5; V22 6.5,-2.5; V23 7.5,-2.5; V24 8.5,-2.5; V25 9.5,-2.5; V26 10.5,-2.5; V27 11.5,-2.5; V28 12.5,-2.5; V29 13.5,-2.5; V30 14.5,-2.5; W1 -14.5,-3.5; W2 -13.5,-3.5; W3 -12.5,-3.5; W4 -11.5,-3.5; W5 -10.5,-3.5; W6 -9.5,-3.5; W7 -8.5,-3.5; W8 -7.5,-3.5; W9 -6.5,-3.5; W10 -5.5,-3.5; W11 -4.5,-3.5; W12 -3.5,-3.5; W13 -2.5,-3.5; W14 -1.5,-3.5; W15 -0.5,-3.5; W16 0.5,-3.5; W17 1.5,-3.5; W18 2.5,-3.5; W19 3.5,-3.5; W20 4.5,-3.5; W21 5.5,-3.5; W22 6.5,-3.5; W23 7.5,-3.5; W24 8.5,-3.5; W25 9.5,-3.5; W26 10.5,-3.5; W27 11.5,-3.5; W28 12.5,-3.5; W29 13.5,-3.5; W30 14.5,-3.5; Y1 -14.5,-4.5; Y2 -13.5,-4.5; Y3 -12.5,-4.5; Y4 -11.5,-4.5; Y5 -10.5,-4.5; Y6 -9.5,-4.5; Y7 -8.5,-4.5; Y8 -7.5,-4.5; Y9 -6.5,-4.5; Y10 -5.5,-4.5; Y11 -4.5,-4.5; Y12 -3.5,-4.5; Y13 -2.5,-4.5; Y14 -1.5,-4.5; Y15 -0.5,-4.5; Y16 0.5,-4.5; Y17 1.5,-4.5; Y18 2.5,-4.5; Y19 3.5,-4.5; Y20 4.5,-4.5; Y21 5.5,-4.5; Y22 6.5,-4.5; Y23 7.5,-4.5; Y24 8.5,-4.5; Y25 9.5,-4.5; Y26 10.5,-4.5; Y27 11.5,-4.5; Y28 12.5,-4.5; Y29 13.5,-4.5; Y30 14.5,-4.5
